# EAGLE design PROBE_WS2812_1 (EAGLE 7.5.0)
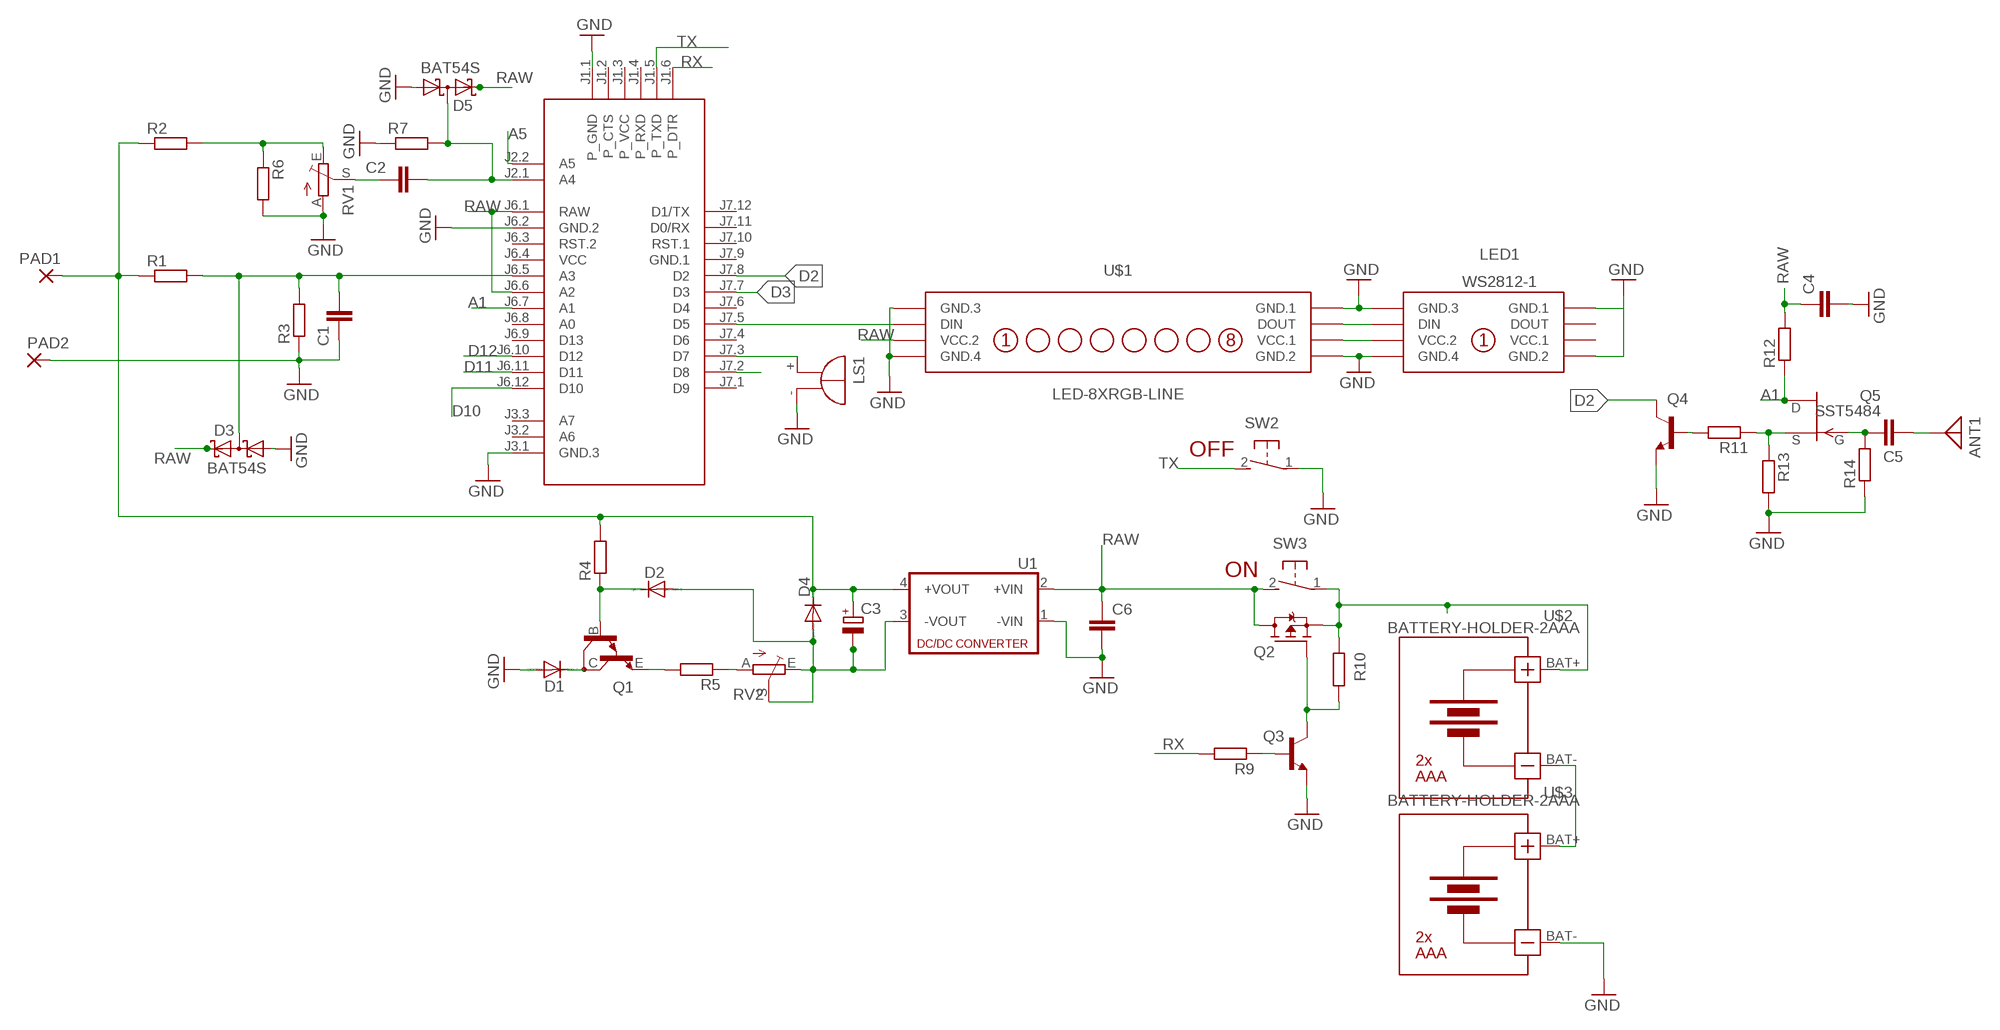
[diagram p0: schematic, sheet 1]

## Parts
ANT1  ANTENNA  [PAD-01]
ARD1  ARDUINO-PRO-MINI-3.3V  [ARDUINO-PRO-MINI]
C1  C-EUC1206  [C1206]
C2  C-EUC1206  [C1206]
C3  CPOL-EUC/6032-28R  [C/6032-28R]
C4  C-EUC0805  [C0805]
C5  C-EUC0805  [C0805]
C6  C-EUC0805  [C0805]
D1  CGRM4007-G  [SOD-123_MINI-SMA]
D2  CGRM4007-G  [SOD-123_MINI-SMA]
D3  BAT54S  [SOT23]
D4  CGRM4001-G  [SOD-123_MINI-SMA]
D5  BAT54S  [SOT23]
LED1  WS2812-1  [WS2812-1]
LS1  BMT1205XH7.5  [BMT1205XH7.5]
PAD1  3,81/1,1  [3,81/1,1]
PAD2  3,81/1,1  [3,81/1,1]
Q1  BDV65  [SOT93]
Q2  STR2P3LLH6  [SOT23]
Q3  BC817-16LT1SMD  [SOT23-BEC]
Q4  BC817-16LT1SMD  [SOT23-BEC]
Q5  SST5484  [SOT23]
R1  R-EU_R2512  [R2512]
R2  R-EU_R2512  [R2512]
R3  R-EU_R2512  [R2512]
R4  R-EU_R2512  [R2512]
R5  R-EU_R2512  [R2512]
R6  R-EU_R2512  [R2512]
R7  R-EU_R0805  [R0805]
R9  R-EU_R0805  [R0805]
R10  R-EU_R0805  [R0805]
R11  R-EU_R0805  [R0805]
R12  R-EU_R0805  [R0805]
R13  R-EU_R0805  [R0805]
R14  R-EU_R0805  [R0805]
RV1  TRIM_EU-CT6  [CT6]
RV2  TRIM_EU-CT6  [CT6]
SW2  31-XX  [B3F-31XX]
SW3  31-XX  [B3F-31XX]
U1  NME  [NME]
U$1  LED-8XRGB-LINE  [LED-8XRGB-LINE]
U$2  BATTERY-HOLDER-2AAA  [BATTERY-HOLDER-2AAA]
U$3  BATTERY-HOLDER-2AAA  [BATTERY-HOLDER-2AAA]

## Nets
A1: ARD1.J6.7(A1) Q5.2(D) R12.1
A3: ARD1.J6.5(A3) C1.2 D3.3(C1A2) R1.2 R3.2
A5: ARD1.J2.2(A5)
BAT: Q2.3(S) R10.2 SW3.1(P) U$2.BAT+
D2: ARD1.J7.8(D2) Q4.C
D3: ARD1.J7.7(D3)
D10: ARD1.J6.12(D10)
D11: ARD1.J6.11(D11)
D12: ARD1.J6.10(D12)
GND: ARD1.J1.1(P_GND) ARD1.J3.1(GND.3) ARD1.J6.2(GND.2) C1.1 C4.2 C6.2 D1.A D3.1(A1) D5.1(A1) LED1.A.1(GND.1) LED1.A.4(GND.2) LED1.B.1(GND.3) LED1.B.4(GND.4) LS1.- PAD2.1(P) Q3.E Q4.E R3.1 R6.2 R7.1 R13.2 R14.1 RV1.A SW2.1(P) U1.1(-VIN) U$1.A.1(GND.1) U$1.A.4(GND.2) U$1.B.1(GND.3) U$1.B.4(GND.4) U$3.BAT-
N$1: R2.2 R6.1 RV1.E
N$2: Q4.B R11.2
N$3: Q5.3(S) R11.1 R13.1
N$4: ARD1.J2.1(A4) C2.2 D5.3(C1A2) R7.2
N$5: ARD1.J7.3(D7) LS1.+
N$6: ARD1.J7.2(D8)
N$7: ANT1.1 C5.2
N$8: Q1.E R5.2
N$9: R5.1 RV2.A
N$10: C3.- D2.A D4.A RV2.E RV2.S U1.3(-VOUT)
N$11: LED1.B.2(DIN) U$1.A.2(DOUT)
N$12: D1.C Q1.C
N$13: C5.1 Q5.1(G) R14.2
N$14: ARD1.J7.5(D5) U$1.B.2(DIN)
N$15: LED1.B.3(VCC.2) U$1.A.3(VCC.1)
N$16: Q2.2(G) Q3.C R10.1
N$18: Q3.B R9.1
N$20: D2.C Q1.B R4.1
N$21: U$2.BAT- U$3.BAT+
N$23: C2.1 RV1.S
N$24: C3.+ D4.C PAD1.1(P) R1.1 R2.1 R4.2 U1.4(+VOUT)
RAW: ARD1.J6.1(RAW) ARD1.J6.6(A2) C4.1 C6.1 D3.2(C2) D5.2(C2) Q2.1(D) R12.2 SW3.2(S) U1.2(+VIN) U$1.B.3(VCC.2)
RX: ARD1.J1.6(P_DTR) R9.2
TX: ARD1.J1.5(P_TXD) SW2.2(S)
Unconnected: ARD1.J1.2(P_CTS) ARD1.J1.3(P_VCC) ARD1.J1.4(P_RXD) ARD1.J3.2(A6) ARD1.J3.3(A7) ARD1.J6.3(RST.2) ARD1.J6.8(A0) ARD1.J6.9(D13) ARD1.J7.1(D9) ARD1.J7.4(D6) ARD1.J7.6(D4) ARD1.J7.10(RST.1) ARD1.J7.11(D0/RX) ARD1.J7.12(D1/TX) LED1.A.2(DOUT)

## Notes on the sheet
- OFF
- ON

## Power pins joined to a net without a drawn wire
GND.1: ARD1.J7.9(GND.1)
VCC: ARD1.J6.4(VCC)
VCC.1: LED1.A.3(VCC.1)

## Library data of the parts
ANT1 = discrete:ANTENNA: Antenna
ARD1 = diy-modules:ARDUINO-PRO-MINI-*: Arduino Pro Mini and compatible devices More details available here: https://www.arduino.cc/en/Main/ArduinoBoardProMini Click here to find device on ebay.com
C1 C2 C4-C6 = rcl:C-EU: CAPACITOR, European symbol
C3 = rcl:CPOL-EU: POLARIZED CAPACITOR, European symbol
D1 D2 D4 = diode:CGRM400*-G: Molded plasitc,JEDEC SOD-123/Mini SMA
D3 D5 = diode:BAT54S: Schottky Diodes Pin connection corrected 2011-05-04 Source: Fairchild .. BAT54.pdf
LED1 = diy-modules:WS2812-1
LS1 = buzzer:BMT1205XH7.5: MAGNETIC TRANSDUCER; OC_FARNELL: unknown; OC_NEWARK: unknown
PAD1 PAD2 = wirepad:3,81/1,1: THROUGH-HOLE PAD
Q1 = transistor:BDV65: NPN BIPOLAR DARLINGTON TRANSISTOR
Q2 = transistor-fet:STR2P3LLH6
Q3 Q4 = transistor-npn:BC817*: NPN Transistor
Q5 = transistor-fet:?548*: N-Channel JFETs Source: VISHAY 2N5484.pdf Compatible: TO92 2N5245 J304 J305 U310 J308 J309 J310 TO72 2N4416 2N4416A 2N3823 2N4351 3N169 3N170 3N171 MFE3002 TO18 2N3796 2N3797 MFE825 Source: Motorola European Master Guide Pacge 3-59
R1-R7 R9-R14 = rcl:R-EU_: RESISTOR, European symbol
RV1 RV2 = pot:TRIM_EU-: POTENTIOMETER
SW2 SW3 = switch-omron:31-XX: OMRON SWITCH; MPN: B3F-3100; OC_FARNELL: 959704; OC_NEWARK: 36M3582
U1 = dc-dc-converter:NME: DC-DC CONVERTER; MF: C & D TECHNOLOGIES, INC; MPN: NME1205D; OC_FARNELL: 1021466; OC_NEWARK: 98B8198
U$1 = diy-modules:LED-8XRGB-LINE: 8 LEDs RGB Line Display based on WS2812B More details about controlling WS2812B RGB LEDs are available here: https://learn.sparkfun.com/tutorials/ws2812-breakout-hookup-guide Click here to find device on ebay.com
U$2 U$3 = diy-modules:BATTERY-HOLDER-2AAA: Battery Holder 2 x AAA

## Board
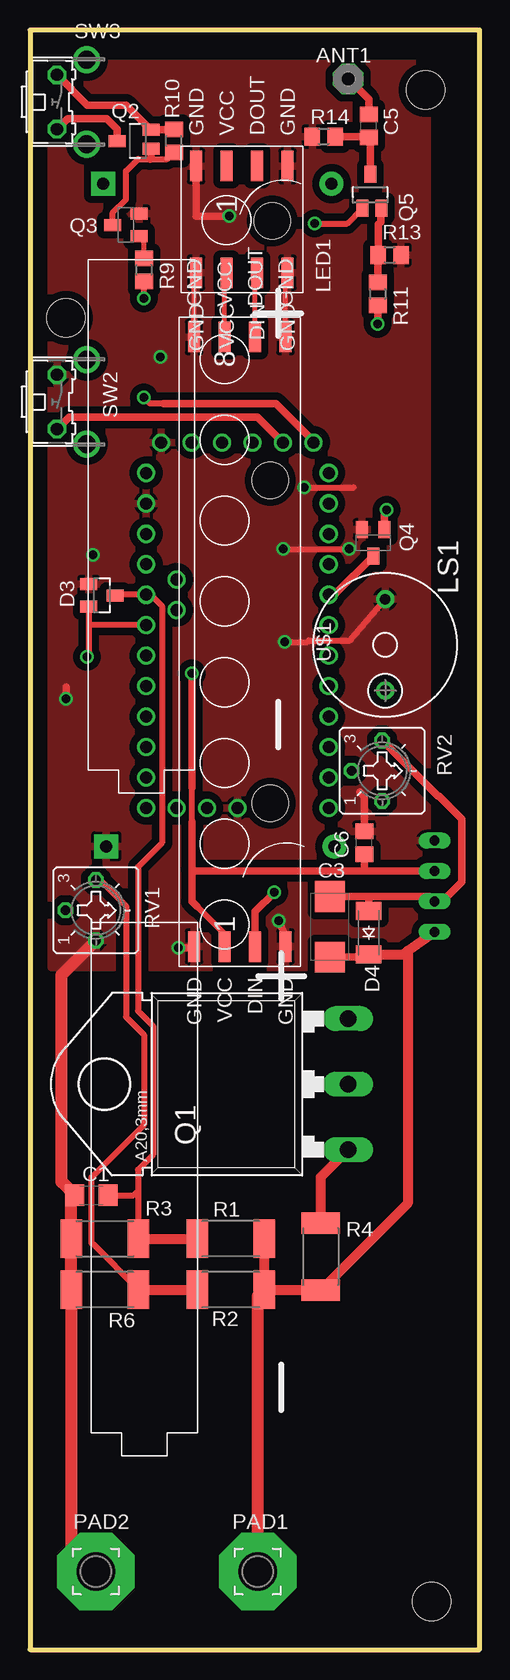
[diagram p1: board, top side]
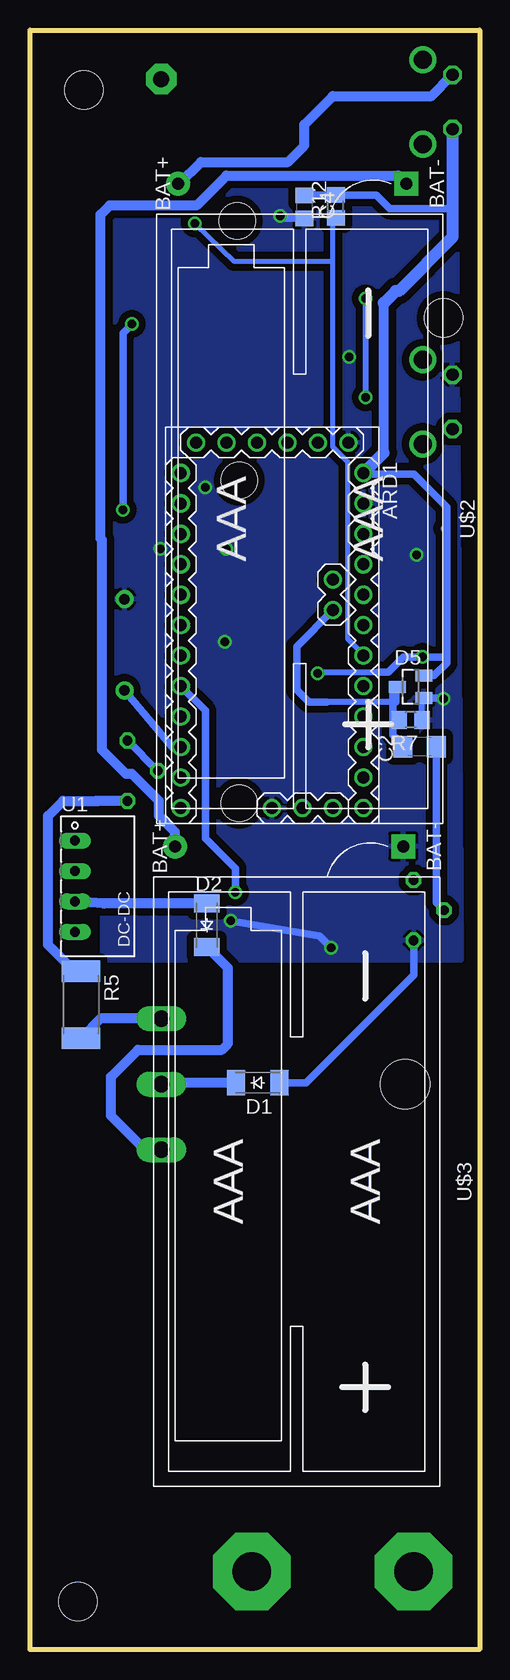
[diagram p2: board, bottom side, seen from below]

Size 37.5 x 135 mm. Coordinates in mm from the lower left corner, seen from the top.
Outline: 0,0 37.5,0 37.5,135 0,135 0,0
Copper layers (1*16): Top 0.035mm / dielectric 1.5mm / Bottom 0.035mm
Design rules "default *": minimum track width 10mil, minimum drill 24mil, track to track 6mil, track to pad 6mil, pad to pad 6mil, via to via 8mil, smd to smd 8mil, copper to edge 20mil, drill to drill 8mil, minimum pad ring 10mil, minimum via ring 8mil, stop-mask expansion 4mil, vias tented up to drill 0mil, thermal gap 10mil
Holes 3.2 mm at 33,130 33.5,4 3,111
bRestrict: area 1.4,37.6 to 11,43.2

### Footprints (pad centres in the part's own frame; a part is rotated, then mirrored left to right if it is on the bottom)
PAD-01 = drill 1.321 pad 2.54 octagon: 1 0,0
ARDUINO-PRO-MINI = drill 1: J1.1 -15.24,6.35; J1.2 -15.24,3.81; J1.3 -15.24,1.27; J1.4 -15.24,-1.27; J1.5 -15.24,-3.81; J1.6 -15.24,-6.35; J2.1 -1.27,5.08; J2.2 -3.81,5.08; J3.1 15.24,0; J3.2 15.24,2.54; J3.3 15.24,5.08; J6.1 -12.7,7.62; J6.2 -10.16,7.62; J6.3 -7.62,7.62; J6.4 -5.08,7.62; J6.5 -2.54,7.62; J6.6 0,7.62; J6.7 2.54,7.62; J6.8 5.08,7.62; J6.9 7.62,7.62; J6.10 10.16,7.62; J6.11 12.7,7.62; J6.12 15.24,7.62; J7.1 15.24,-7.62; J7.2 12.7,-7.62; J7.3 10.16,-7.62; J7.4 7.62,-7.62; J7.5 5.08,-7.62; J7.6 2.54,-7.62; J7.7 0,-7.62; J7.8 -2.54,-7.62; J7.9 -5.08,-7.62; J7.10 -7.62,-7.62; J7.11 -10.16,-7.62; J7.12 -12.7,-7.62
C1206 = smd 1.6 x 1.8: 1 -1.4,0; 2 1.4,0
C/6032-28R = smd 2.55 x 2.5: + 2.525,0; - -2.525,0
C0805 = smd 1.3 x 1.5: 1 -0.95,0; 2 0.95,0
SOD-123_MINI-SMA = smd 1.5 x 2.1: A 1.8,0; C -1.8,0
SOT23 = smd 1 x 1.4: 1 -0.95,-1.1; 2 0.95,-1.1; 3 0,1.1
WS2812-1 = smd 2.54 x 1.016: A.1 -10.16,-1.27; A.2 -10.16,-3.81; A.3 -10.16,-6.35; A.4 -10.16,-8.89; B.1 -1.27,-1.27; B.2 -1.27,-3.81; B.3 -1.27,-6.35; B.4 -1.27,-8.89 | hole 3: -5.588,-2.54
BMT1205XH7.5 = drill 0.9 pad 1.5: + 3.8,0; - -3.8,0
3,81/1,1 = drill 3.2 pad 6.452 octagon: 1 0,0
SOT93 = drill 1.397 long: B -5.461,-10.16; C 0,-10.16; E 5.461,-10.16 | hole 4.115: 0,10.16
SOT23' = smd 1 x 1.4: 1 0,1.735; 2 -0.632,-1.1; 3 0.95,-1.1
SOT23-BEC = smd 1 x 1.4: B -0.95,-1.1; C 0,1.1; E 0.95,-1.1
R2512 = smd 1.8 x 3.2: 1 -2.8,0; 2 2.8,0
R0805 = smd 1.3 x 1.5: 1 -0.95,0; 2 0.95,0
CT6 = drill 0.813 octagon: A 2.515,0; E -2.515,0; S 0,-2.54
B3F-31XX = drill 1.016 octagon: 1 -2.261,-1.245; 2 2.261,-1.245 | drill 1.499 pad 2.159: 3 -3.505,1.245; 4 3.505,1.245
NME = drill 0.813 long: 1 0,3.81; 2 0,1.27; 3 0,-1.27; 4 0,-3.81
LED-8XRGB-LINE = smd 2.54 x 1.016: A.1 -25.4,3.81; A.2 -25.4,1.27; A.3 -25.4,-1.27; A.4 -25.4,-3.81; B.1 25.4,3.81; B.2 25.4,1.27; B.3 25.4,-1.27; B.4 25.4,-3.81 | hole 3: -13.462,2.54; 13.462,2.54
BATTERY-HOLDER-2AAA = drill 1 pad 2: BAT+ -27.94,-10.16 | drill 1 pad 2 square: BAT- -27.94,8.89

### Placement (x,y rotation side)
ANT1  26.55,130.91 0 top
ARD1  17.3,85.38 270 bottom
C1  5.12,37.88 0 top
C2  5,75.25 180 bottom
C3  25,60.25 270 top
C4  14.62,120.25 270 bottom
C5  28.25,127 90 top
C6  27.88,67.25 90 top
D1  18.5,47.25 0 bottom
D2  22.75,60.38 90 bottom
D3  6,87.88 270 top
D4  28.25,59.75 90 top
D5  5.75,80.25 90 bottom
LED1  22.75,113.5 270 top
LS1  29.62,83.75 270 top
PAD1  19,6.5 0 top
PAD2  5.5,6.5 0 top
Q1  16.38,47.12 90 top
Q2  STR2P3LLH6  [SOT23']  9,125.75 90 top
Q3  8,118.75 90 top
Q4  28.62,92.25 180 top
Q5  SST5484  [SOT23']  28.38,121.25 0 top
R1  16.75,34.25 180 top
R2  16.75,30 180 top
R3  6.25,34.25 0 top
R4  24.25,32.75 270 top
R5  33.25,53.75 270 bottom
R6  6.25,30 180 top
R7  5.75,77.5 180 bottom
R9  9.5,115 270 top
R10  12,125.75 90 top
R11  29,113 270 top
R12  12,120.3 90 bottom
R13  30,116.25 0 top
R14  24.5,126.12 0 top
RV1  5.5,61.62 270 top
RV2  29.38,73.25 270 top
SW2  3.5,104 270 top
SW3  3.5,129 270 top
U1  33.75,63.62 0 bottom
U$1  17.5,84 270 top
U$2  15,94.25 270 bottom
U$3  15.25,39 270 bottom

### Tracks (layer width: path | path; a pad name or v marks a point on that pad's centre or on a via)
A1  (via drill 0.7)
  Top 0.5: v23.75,118.88 26.47,118.88 Q5.2
  Bottom 0.406: ARD1.J6.7 9.68,82.93 11,84.25 11,99 12.25,100.25 12.25,115.75 | v23.75,118.88 20.5,115.75 12.25,115.75 | 12.25,115.75 12.25,119.1 R12.1
A3
  Top 0.5: 9,38.25 9,40 10.25,41.25 10.25,52 9,53.25 9,65.25 11,67.25 11,87 10.08,87.92 ARD1.J6.5 7.14,87.92 D3.3 | 9,38.25 9,34.3 R3.2 | C1.2 8.62,37.88 9,38.25
  Top 0.813: R3.2 R1.2
BAT
  Top 0.61: SW3.1 4.77,128.75 8,128.75 10.05,126.7 Q2.3 R10.2
  Bottom 0.813: U$2.BAT+ 25.06,122.19 23.25,124 16,124 14.62,125.38 14.62,127.12 12.25,129.5 4.02,129.5 SW3.1
D2
  Top 0.61: ARD1.J7.8 25.39,87.92 Q4.C
GND  (via drill 0.7)
  Top 0.406: U$1.A.1 21.31,114.6 LED1.B.1 | U$1.A.4 13.69,114.6 LED1.B.4 | 8.93,119.88 Q3.E
  Top 0.5: v21.25,84 23.12,84 23.25,84.12 26.68,84.12 LS1.- | v22.88,96.88 27,96.88 | 21,91.75 26.5,91.75
  Top 0.61: U$1.B.1 21.31,59.44 v20.75,60.75 | v12.38,58.5 13.59,58.5 U$1.B.4 | v16.62,119.5 13.86,119.5 LED1.A.4 | C6.2 27.88,71.12 27.5,71.5 | v3,79.25 3,80.25
  Top 1.016: RV1.A 2.62,56.23 2.62,38.98 C1.1 3.45,37.6 R3.1 R6.2 3.45,8.55 PAD2.1
  Bottom 0.5: R7.1 4.8,79.15 D5.1
  Bottom 0.61: D1.A 14.5,47.25 5.5,56.25 RV1.A | v20.75,60.75 13.38,59.5 v12.38,58.5 | C4.2 16.62,119.3 v16.62,119.5 | D5.1 3.05,79.3 v3,79.25
  other vias: 10.88,107.75 21.12,91.75 5.25,91.25 26.62,91.75
  pour Bottom (isolate 0.61): 2,132.5 31.5,132.5 31.5,57.5 1.5,57.5
  pour Top (isolate 0.61): 1.75,132.25 33.12,132.25 33.12,56.88 1.75,56.88
N$1
  Top 0.5: RV1.E 5.86,64.14 8,62 8,52.75 9.5,51.25 9.5,43.75 5.12,39.38 5.12,33.88 5.2,33.8 5.25,33.8 R6.1
  Top 0.813: R6.1 R2.2
N$2  (via drill 0.7)
  Top 0.61: Q4.B 29.57,94.83 v29.75,95 | v29,110.5 R11.2
  Bottom 0.61: v29.75,95 29.75,109.75 v29,110.5
N$3
  Top 0.61: R11.1 29,116.2 R13.1 29.05,118.8 29.25,119 29.25,120.08 Q5.3
N$4
  Bottom 0.5: R7.2 6.75,77.5 7.25,78 | 7,79 12.75,79
  Bottom 0.61: C2.2 6.4,75.4 7.25,76.25 7.25,78 7.25,79.85 D5.3 6.85,80.15 7,80 7,79 | 12.75,79 14.25,79 15.25,80 15.25,83.62 ARD1.J2.1
N$5
  Bottom 0.61: ARD1.J7.3 25.64,75.22 LS1.+
N$7
  Top 0.61: C5.2 28.25,129.21 ANT1.1
N$8
  Bottom 0.813: Q1.E 31.61,52.59 R5.2
N$9
  Bottom 0.813: RV2.A 31.75,70.73 | 31.75,70.73 32.02,70.73 | R5.1 33.25,56.75 34,56.75 36,58.75 36,69.5 34.75,70.75 31.77,70.75 31.75,70.73
N$10
  Top 0.61: C3.- 27.02,62.77 | C3.- 28.12,62.77 28.25,62.65 D4.A | U1.3 32.86,62.35 | RV2.E 34,71.14 34.11,71.14 36,69.25 36,64 34.5,62.5 33.9,62.5 U1.3 | C3.- 33.33,62.77 U1.3
  Bottom 0.61: RV2.S 26.86,73.25 RV2.E
  Bottom 0.813: D2.A 31.32,62.17 U1.3
N$11
  Top 0.406: U$1.A.2 18.77,114.6 LED1.B.2
N$12
  Bottom 0.813: D1.C 26.41,47.25 Q1.C
N$13
  Top 0.61: Q5.1 28.38,125.92 C5.1 28.18,126.12 R14.2
N$14  (via drill 0.7)
  Top 0.61: U$1.B.2 18.77,61.52 v20.38,63.12
  Bottom 0.61: v20.38,63.12 20.38,65.12 22.88,67.62 22.88,78.25 ARD1.J7.5
N$15
  Top 0.406: U$1.A.3 16.23,114.6 LED1.B.3
N$16
  Top 0.5: Q3.C 6.9,119.78 8,120.88 8,123.25 9,124.25 10,124.25 11.45,124.25 R10.1
  Top 0.61: Q2.2 10.1,124.35 10,124.25
N$18
  Top 0.406: R9.1 9.5,117.4 Q3.B
N$20
  Top 0.813: R4.1 24.25,39.38 Q1.B
  Bottom 0.813: Q1.B 27.91,41.66 30.75,44.5 30.75,47.75 28.5,50 21.5,50 21,50.5 21,56.83 D2.C
N$21
  Bottom 0.813: U$2.BAT- 6.79,122.88 21.12,122.88 23.62,120.38 30.88,120.38 31.62,119.62 31.62,92.62 31.5,92.5 31.5,75 29.5,73 29,73 26.75,70.75 26.75,69.5 25.41,68.16 U$3.BAT+
N$23
  Bottom 0.61: C2.1 3.6,62.27 RV1.S
N$24
  Top 0.61: C3.+ 28.02,57.73 D4.C
  Top 0.813: R1.1 R2.1 24.2,30 R4.2 31.5,37.2 31.5,58.25 | U1.4 31.5,58.25 | D4.C 31.2,57.95 31.5,58.25
  Top 1.016: PAD1.1 19,29.45 R2.1
RAW  (via drill 0.7)
  Top 0.5: U$1.B.3 16.23,59.65 13.94,61.94 | 13.5,69 13.5,71.88 | D3.2 4.9,85.38 | 4.9,85.38 4.9,82.9 v4.75,82.75 | ARD1.J6.6 4.9,85.38
  Top 0.61: 13.5,71.88 v13.5,81.38 | U1.2 27.75,64.9 | 27.75,64.9 13.61,64.9 13.5,65 | Q2.1 7.26,126.73 6.38,127.62 3.14,127.62 SW3.2 | C6.1 27.88,65.02 27.75,64.9 | 13.5,69 13.5,65 | 13.5,65 13.5,62.38 13.94,61.94
  Bottom 0.5: v13.5,81.38 13.38,81.38 13.25,81.5 8.5,81.5
  Bottom 0.61: D5.2 3.8,81.2 2.75,82.25 2.75,82.75 | 2.75,82.75 2.75,93.25 | 2.75,93.25 2.75,95.25 5.5,98 9.6,98 ARD1.J6.1 | 2.95,93.45 2.75,93.25 | 2.75,82.75 v4.75,82.75 6.38,82.75 7.62,81.5 8.5,81.5 | 2.25,119.75 2.63,120.12 7.5,120.12 8.62,121.25 R12.2 14.57,121.25 C4.1
  Bottom 0.813: 8,99.76 8,112.25
  Bottom 1.016: SW3.2 2.25,119.75 2.25,117.75 6.75,113.25 7,113.25 8,112.25 | 8,99.76 ARD1.J6.1
RX  (via drill 0.7)
  Top 0.5: 11.12,103.88 10,103.88 v9.5,104.38 | v9.5,112.62 R9.2
  Top 0.61: ARD1.J1.6 23.65,100.72 20.5,103.88 11.12,103.88 | 9.62,113.92 R9.2
  Bottom 0.5: v9.5,104.38 v9.5,112.62
TX
  Top 0.61: SW2.2 2.25,101.75 3.25,102.75 18.98,102.75 ARD1.J1.5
